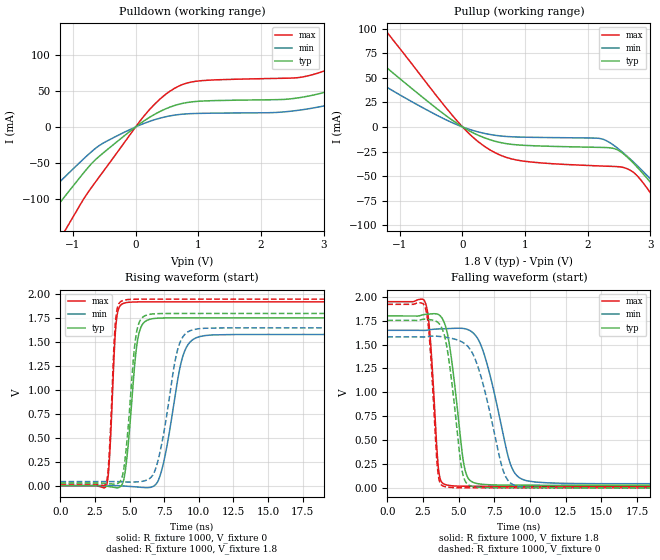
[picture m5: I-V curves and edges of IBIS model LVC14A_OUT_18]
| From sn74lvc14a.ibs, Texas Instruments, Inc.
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[Model]   LVC14A_OUT_18
Model_type  Output
Vref =   0
Rref =   1000
Cref =   30p
Vmeas =   0.9
| variable   typ   min   max
C_comp   8.26pF   4.12pF   14.97pF
| C_pullup   6.94pF   4.12pF   8.26pF
| C_pulldown   9.57pF   4.62pF   14.97pF
[Temperature Range]   40   100   -40
| Ambient temperature   25   85   -40
[Voltage range]   1.8   1.65   1.95
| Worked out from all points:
|   slope of the pulldown table from 0 to 0.27 V, typ, clamps not added: 17.1 ohm
|   slope of the pullup table from 0 to 0.27 V, typ, clamps not added: 29.9 ohm
|   rising waveform, R_fixture 1000, V_fixture 0: 20-80 % time 619ps typ, 1.12ns min, 360ps max; typ from 0 V to 1.75 V
|   falling waveform, R_fixture 1000, V_fixture 1.8: 20-80 % time 828ps typ, 1.48ns min, 466ps max; typ from 1.8 V to 0.027 V
|   rising waveform, R_fixture 1000, V_fixture 1.8: 20-80 % time 604ps typ, 1.11ns min, 354ps max; typ from 0.027 V to 1.8 V
|   falling waveform, R_fixture 1000, V_fixture 0: 20-80 % time 822ps typ, 1.51ns min, 462ps max; typ from 1.75 V to 0 V
[Pulldown]
| LVC14A_OUT_18
|   Voltage   I(typ)   I(min)   I(max)
-5.5V     -562.8mA   -456mA     -714.6mA
-1.87V    -176.7mA   -133mA     -245.9mA
-1.485V   -135.1mA   -99.63mA   -194.2mA
-1.07V    -89.57mA   -64.08mA   -135.1mA
-570mV    -39.87mA   -25.16mA   -67.84mA
70mV      4.491mA    2.617mA    8.125mA
615mV     29.45mA    16.27mA    53.12mA
2.815V    43.69mA    25.92mA    72.1mA
4.325V    93.52mA    64.21mA    142.7mA
5.155V    134.5mA    96.03mA    199.6mA
6.155V    191.3mA    141.3mA    276.1mA
11V       510.2mA    405.2mA    689.3mA
[Pullup]
| LVC14A_OUT_18
|   Voltage   I(typ)   I(min)   I(max)
-5.5V     324.9mA    249.5mA    454.8mA
-2.68V    143.9mA    103mA      216.3mA
-2.015V   104.9mA    73.15mA    161.8mA
-1.32V    66.21mA    44.72mA    105.6mA
360mV     -11.3mA    -6.711mA   -20.18mA
980mV     -18.71mA   -10.42mA   -34.85mA
2.465V    -23.03mA   -21.11mA   -40.36mA
2.81V     -42.39mA   -40.68mA   -51.19mA
3.355V    -85.4mA    -77.55mA   -102.6mA
3.555V    -102.9mA   -92.26mA   -124.5mA
3.77V     -122.5mA   -108.6mA   -148.9mA
11V       -881.1mA   -746.6mA   -1.074A
[Ramp]
| LVC14A_OUT_18
| variable   typ   min   max
dV/dt_r   1.07/6.30E-10   0.96/1.14E-09   1.17/3.68E-10
dV/dt_f   1.08/8.45E-10   0.98/1.51E-09   1.18/4.80E-10
R_load = 1000
[Rising Waveform]
| LVC14A_OUT_18
R_fixture =   1000
C_fixture =   0
L_fixture =   0
V_fixture =   0
V_fixture_min = 0
V_fixture_max = 0
|   Time   V(typ)   V(min)   V(max)
0s        194.2pV    4.892nV    16.26pV
3.35ns    -5.394mV   239.6uV    11.51mV
4.025ns   -21.63mV   12.13uV    1.698V
4.64ns    110.6mV    -4.369mV   1.909V
5.57ns    1.515V     -14.23mV   1.921V
6.49ns    1.74V      -18.27mV   1.922V
7.385ns   1.753V     198mV      1.922V
8.88ns    1.754V     1.368V     1.922V
10.09ns   1.754V     1.559V     1.922V
50ns      1.754V     1.581V     1.922V
[Falling Waveform]
| LVC14A_OUT_18
R_fixture =   1000
C_fixture =   0
L_fixture =   0
V_fixture =   1.8
V_fixture_min = 1.65
V_fixture_max = 1.95
|   Time   V(typ)   V(min)   V(max)
0s        1.8V       1.65V      1.95V
2.685ns   1.817V     1.649V     1.929V
3ns       1.821V     1.656V     1.582V
3.585ns   1.815V     1.664V     197mV
4.13ns    1.665V     1.667V     31.47mV
5.38ns    232.1mV    1.668V     17.09mV
6.215ns   47.58mV    1.589V     16.42mV
8.62ns    28.22mV    250.4mV    16.27mV
9.77ns    27.46mV    74.43mV    16.27mV
50ns      27.13mV    42.42mV    16.27mV
[Rising Waveform]
| LVC14A_OUT_18
R_fixture =   1000
C_fixture =   0
L_fixture =   0
V_fixture =   1.8
V_fixture_min = 1.65
V_fixture_max = 1.95
|   Time   V(typ)   V(min)   V(max)
0s        27.13mV    42.42mV    16.27mV
3.315ns   22.91mV    42.52mV    33.9mV
3.995ns   17.5mV     42.18mV    1.739V
4.59ns    186.3mV    39.05mV    1.939V
5.465ns   1.571V     38.81mV    1.949V
6.325ns   1.787V     63.74mV    1.95V
7.155ns   1.799V     323.6mV    1.95V
8.52ns    1.8V       1.446V     1.95V
9.61ns    1.8V       1.631V     1.95V
50ns      1.8V       1.65V      1.95V
[Falling Waveform]
| LVC14A_OUT_18
R_fixture =   1000
C_fixture =   0
L_fixture =   0
V_fixture =   0
V_fixture_min = 0
V_fixture_max = 0
|   Time   V(typ)   V(min)   V(max)
0s        1.754V     1.581V     1.922V
2.66ns    1.766V     1.58V      1.884V
2.97ns    1.762V     1.587V     1.526V
3.535ns   1.733V     1.587V     176mV
4.01ns    1.591V     1.579V     14.1mV
5.215ns   196.8mV    1.529V     755.6uV
5.935ns   15.89mV    1.418V     160.9uV
8.11ns    837.3uV    183mV      2.286uV
9.115ns   288.8uV    18.49mV    344.3nV
50ns      4.829nV    8.848nV    1.448nV
